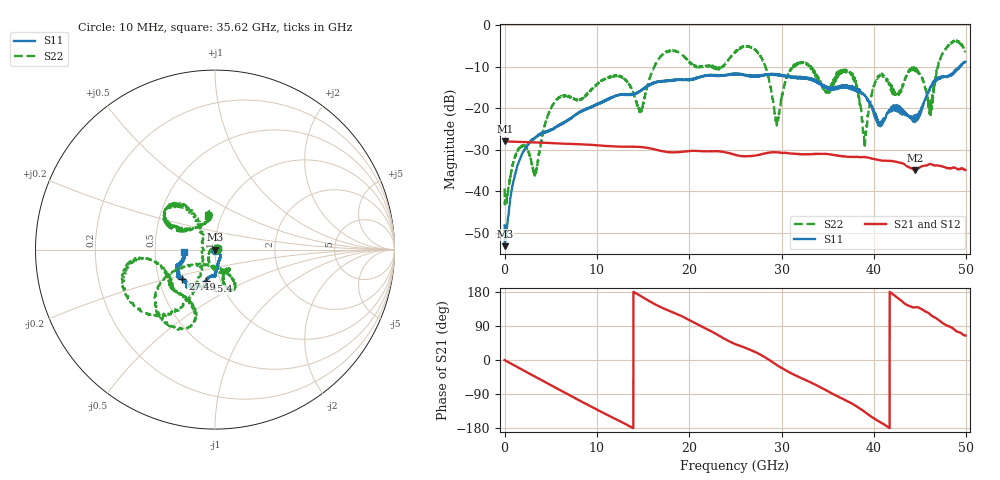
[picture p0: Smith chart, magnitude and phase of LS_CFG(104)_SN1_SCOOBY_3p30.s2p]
!Keysight Technologies,N5245B,MY58422026,A.13.80.08
!Date: Thursday, March 19, 2020 23:59:47
!Correction: S11(Full 2 Port(1,2))
!S21(Full 2 Port(1,2))
!S12(Full 2 Port(1,2))
!S22(Full 2 Port(1,2))
!S2P File: Measurements: S11, S21, S12, S22:
# Hz S DB R 50.0
!freq dBS11 angS11 dBS21 angS21 dBS12 angS12 dBS22 angS22
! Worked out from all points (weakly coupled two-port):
!   4991 points, 10 MHz to 49.91 GHz, reference 50 ohm
!   highest |S21| = -27.99 dB at 20 MHz (marker M1); lowest = -35.0 dB at 44.44 GHz (marker M2)
!   lowest |S11| = -53.2 dB at 30 MHz (marker M3), VSWR 1.00, Z = 50.2 - j0.0279 ohm
!   |S11| at or under -10 dB: start of sweep to 49.25 GHz; 49.28367 GHz to 49.34349 GHz (59.82 MHz wide, 0.121 % of centre)
!   |S22| runs from -43.2 to -3.7 dB; largest |S21 - S12| = 0.00039
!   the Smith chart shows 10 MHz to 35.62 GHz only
!   S11 on the Smith chart (normalised r, x): 10 MHz: 1.01, -0.01; 15.4 GHz: 0.86, -0.31; 27.49 GHz: 0.66, -0.23; 35.62 GHz: 0.71, -0.02
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1e7  -48.22 -47.5  -28.00 -0.3  -27.99 -0.3  -39.32 4.7
2e7  -52.76 -21.8  -27.99 -0.3  -27.98 -0.4  -42.02 -2.7
3e7  -53.22 -7.3  -28.00 -0.5  -28.00 -0.5  -42.34 -9.6
2.24e9  -29.63 -40.5  -28.17 -29.9  -28.15 -29.9  -28.99 23.5
3.31e9  -27.04 -49.2  -28.25 -44.0  -28.24 -43.9  -35.78 130.7
5.27e9  -24.91 -61.6  -28.42 -69.9  -28.42 -69.9  -19.02 -91.6
8.33e9  -20.85 -80.3  -28.71 -109.7  -28.70 -109.6  -17.78 -64.2
1.54e10  -14.79 -105.2  -29.53 159.4  -29.52 159.4  -15.51 -146.3
1.665e10  -13.67 -105.7  -30.14 142.7  -30.13 142.7  -8.30 -145.6
2.496e10  -11.83 -127.7  -31.20 42.2  -31.19 42.4  -6.56 -170.8
2.749e10  -12.28 -138.4  -31.27 17.1  -31.28 17.3  -6.65 -127.7
2.948e10  -11.87 -142.5  -30.62 -13.0  -30.62 -12.6  -23.84 -176.8
3.328e10  -13.05 -158.7  -31.05 -60.7  -31.05 -60.3  -10.59 153.2
3.562e10  -15.29 -175.1  -31.24 -90.7  -31.18 -90.2  -14.36 99.5
3.77e10  -15.54 175.1  -31.72 -116.2  -31.65 -116.3  -12.14 131.6
3.902e10  -16.93 173.9  -31.77 -137.0  -31.74 -137.3  -28.65 -114.6
4.021e10  -22.58 164.6  -32.34 -157.1  -32.33 -157.3  -13.45 -8.6
4.16e10  -20.61 102.7  -32.67 -178.2  -32.70 -178.2  -14.11 22.6
4.444e10  -22.69 47.3  -34.95 139.0  -34.98 139.4  -10.55 -18.2
4.614e10  -14.93 3.5  -33.45 119.3  -33.47 119.3  -21.35 -50.7
4.757e10  -12.36 4.9  -34.16 95.6  -34.16 95.8  -6.26 -80.3
4.991e10  -8.85 -13.7  -34.88 64.5  -34.89 64.7  -6.27 -28.7
